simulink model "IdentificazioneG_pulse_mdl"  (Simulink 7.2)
settings: Solver=ode45  StartTime=0.0  StopTime=100  RelTol=1e-3
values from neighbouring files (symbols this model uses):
  Tp = Tf/3    (= 33.3333333333)    [IdentificazioneG.m]
  Ts = 0.1    [IdentificazioneG.m]
undefined symbols (not defined in the file or in its folder): A
libraries: simulink x1, cstblocks x1

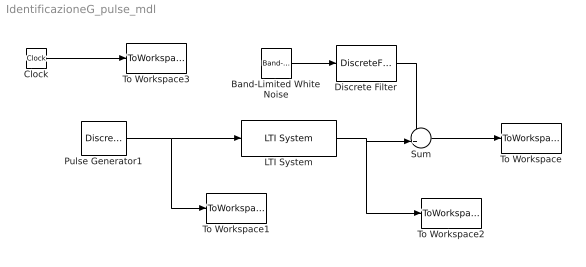
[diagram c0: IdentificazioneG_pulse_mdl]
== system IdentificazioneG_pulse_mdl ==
  Band-Limited White Noise : simulink/Sources/Band-Limited White Noise  SystemSampleTime=-1  Cov=NP  Ts=Ts  seed=[23341]
  Clock : Clock
  Discrete Filter : DiscreteFilter  Denominator=A  SampleTime=Ts
  LTI System : cstblocks/LTI System  SystemSampleTime=-1  sys=G  IC=[]
  Pulse Generator1 : DiscretePulseGenerator  PulseType=Time based  Period=Tp  PulseWidth=50
  Sum : Sum  Inputs=++|  OutDataType=sfix(16)  OutScaling=2^0
  To Workspace : ToWorkspace  VariableName=yn  SampleTime=Ts  SaveFormat=Array
  To Workspace1 : ToWorkspace  VariableName=u  SampleTime=Ts  SaveFormat=Array
  To Workspace2 : ToWorkspace  VariableName=y  SampleTime=Ts  SaveFormat=Array
  To Workspace3 : ToWorkspace  VariableName=time  SampleTime=-1  SaveFormat=Array
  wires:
  Pulse Generator1/1 -> LTI System/1, To Workspace1/1
  Clock/1 -> To Workspace3/1
  Sum/1 -> To Workspace/1
  LTI System/1 -> Sum/2, To Workspace2/1
  Band-Limited White Noise/1 -> Discrete Filter/1
  Discrete Filter/1 -> Sum/1
